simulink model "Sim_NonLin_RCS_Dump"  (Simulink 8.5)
settings: Solver=ode45  StartTime=0.0  StopTime=25*60  FixedStep=Ts  RelTol=1e-3
InitFcn:
  | start2
StopFcn:
  | Pl
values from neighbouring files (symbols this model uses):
  Ave = [    [vehicle_flex34.m]    (also in vehicle_rigid.m)
  Bve = [    [vehicle_flex34.m]    (also in vehicle_rigid.m)
  CB2L = [cpsi, -cphi*spsi,  sphi*spsi;          0,    cphi,      -sphi;          0,    sphi*cpsi,  cphi*cpsi]/cpsi    [Rigbod_Dynam_LVLH.m]    (also in start.m = eye(3); start2.m = eye(3); start3.m = eye(3); start1.m = eye(3))
  com_dir = com_dir/sqrt(com_dir'*com_dir)    [start.m]    (also in start2.m; start3.m; start1.m)
  Cve = [    [vehicle_flex34.m]    (also in vehicle_rigid.m)
  d2r = pi/180    (= 0.0174532925199)    [start.m]    (also in start2.m; start3.m; Dead_Band_DF.m; start1.m)
  Dve = [    [vehicle_flex34.m]    (also in vehicle_rigid.m)
  ini = [wbo; atto; Hco]    [start.m]    (also in start2.m; start3.m; start1.m)
  KshR = 2*Wdot_Lim_RCS/WlimR    [start.m]    (also in start2.m; start3.m; start1.m)
  nt = 12    [start.m]    (also in start2.m; start3.m; start1.m)
  r2d = 180/pi    (= 57.2957795131)    [start.m]    (also in start2.m; start3.m; start1.m)
  thecmd = 20    [start.m]    (also in start2.m; start3.m; start1.m = 0.1)
  Wdot_Lim_RCS = 0.02*d2r    (= 0.000349065850399)    [start.m]    (also in start2.m; start3.m; start1.m)
  Wlim_RCS = 0.6*d2r    (= 0.010471975512)    [start.m]    (also in start2.m; start3.m; start1.m)
  wo = 0.0011    [start.m]    (also in start2.m; start3.m; start1.m)
undefined symbols (not defined in the file or in its folder): Mom_Dump, Phase_Plane, Rigbod_Dynam_LVLH, Wlim

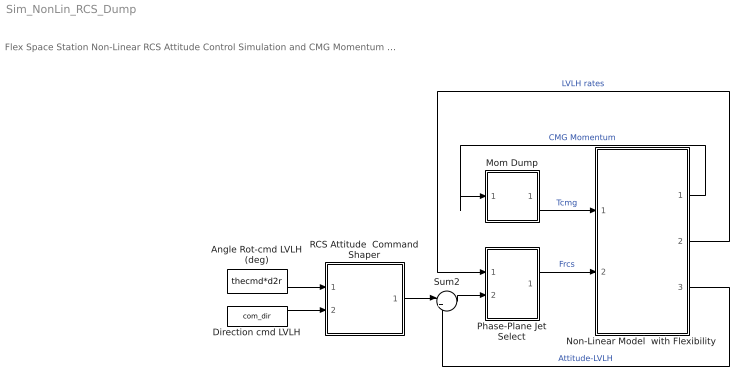
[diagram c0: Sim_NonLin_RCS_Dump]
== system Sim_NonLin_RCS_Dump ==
  note: Flex Space Station Non-Linear RCS Attitude Control Simulation and CMG Momentum Desaturation Mode using RCS
  Angle Rot-cmd LVLH (deg) : Constant  Value=thecmd*d2r
  Direction cmd LVLH : Constant  Value=com_dir
  Mom Dump : Subsystem
  Non-Linear Model  with Flexibility : Subsystem
  Phase-Plane Jet Select : Subsystem
  RCS Attitude  Command Shaper : Subsystem
  Sum2 : Sum  Inputs=|+-
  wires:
  Non-Linear Model  with Flexibility/3(atti) -> Sum2/2  "Attitude-LVLH"
  Non-Linear Model  with Flexibility/1(Hcmg) -> Mom Dump/1(Hcmg)  "CMG Momentum"
  Sum2/1 -> Phase-Plane Jet Select/2(atter)
  Non-Linear Model  with Flexibility/2(w-lv) -> Phase-Plane Jet Select/1(rater)  "LVLH rates"
  Direction cmd LVLH/1 -> RCS Attitude  Command Shaper/2(dir)
  Angle Rot-cmd LVLH (deg)/1 -> RCS Attitude  Command Shaper/1(cmd)
  RCS Attitude  Command Shaper/1(att-cmd) -> Sum2/1
  Phase-Plane Jet Select/1(f(i)) -> Non-Linear Model  with Flexibility/2(Frcs)  "Frcs"
  Mom Dump/1(Tq) -> Non-Linear Model  with Flexibility/1(Tcmg)  "Tcmg"

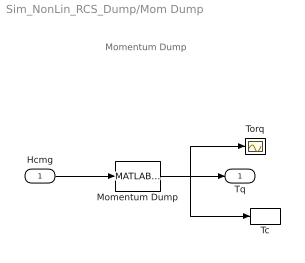
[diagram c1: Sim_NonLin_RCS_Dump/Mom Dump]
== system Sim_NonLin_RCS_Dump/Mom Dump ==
  note: Momentum Dump
  Hcmg : Inport  PortDimensions=3
  Momentum Dump : MATLABFcn  MATLABFcn=Mom_Dump( u(1:3) )  OutputDimensions=3
  Tc : ToWorkspace  VariableName=Tcmg  SampleTime=-1
  Torq : Scope
  Tq : Outport
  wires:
  Momentum Dump/1 -> Tc/1, Torq/1, Tq/1
  Hcmg/1 -> Momentum Dump/1

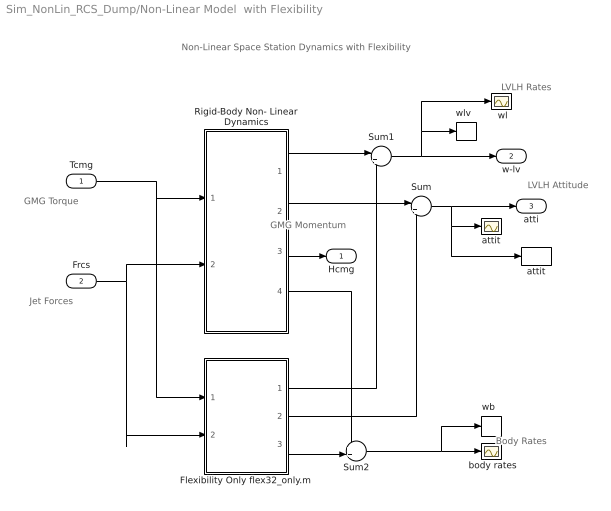
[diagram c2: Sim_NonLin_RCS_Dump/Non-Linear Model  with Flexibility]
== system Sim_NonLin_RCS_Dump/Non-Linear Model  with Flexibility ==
  note: Non-Linear Space Station Dynamics with Flexibility
  note: GMG Torque
  note: Jet Forces
  note: LVLH Rates
  note: LVLH Attitude
  note: Body Rates
  note: GMG Momentum
  Tcmg : Inport
  Frcs : Inport  Port=2
  " attit " : Scope
  " body rates" : Scope
  " wl" : Scope
  Flexibility Only flex32_only.m : Subsystem
  Rigid-Body Non- Linear Dynamics : Subsystem
  Sum : Sum  Inputs=|++
  Sum1 : Sum  Inputs=|++
  Sum2 : Sum  Inputs=++|
  attit : ToWorkspace  VariableName=theta  SampleTime=-1
  "wb  " : ToWorkspace  VariableName=wb  SampleTime=-1
  "wlv  " : ToWorkspace  VariableName=wl  SampleTime=-1
  Hcmg : Outport
  w-lv : Outport  Port=2
  atti : Outport  Port=3
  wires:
  Frcs/1 -> Rigid-Body Non- Linear Dynamics/2(Frcs), Flexibility Only flex32_only.m/2(Frcs)
  Rigid-Body Non- Linear Dynamics/2(atti-lv) -> Sum/1
  Flexibility Only flex32_only.m/2(att) -> Sum/2
  Sum/1 -> atti/1, " attit "/1, attit/1
  Sum1/1 -> w-lv/1, "wlv  "/1, " wl"/1
  Tcmg/1 -> Rigid-Body Non- Linear Dynamics/1(Tcmg), Flexibility Only flex32_only.m/1(Tcmg)
  Rigid-Body Non- Linear Dynamics/1(w-lv) -> Sum1/1
  Flexibility Only flex32_only.m/1(wbf) -> Sum1/2
  Flexibility Only flex32_only.m/3(wb) -> Sum2/2
  Rigid-Body Non- Linear Dynamics/4(wb) -> Sum2/1
  Sum2/1 -> " body rates"/1, "wb  "/1
  Rigid-Body Non- Linear Dynamics/3(Hcmg) -> Hcmg/1

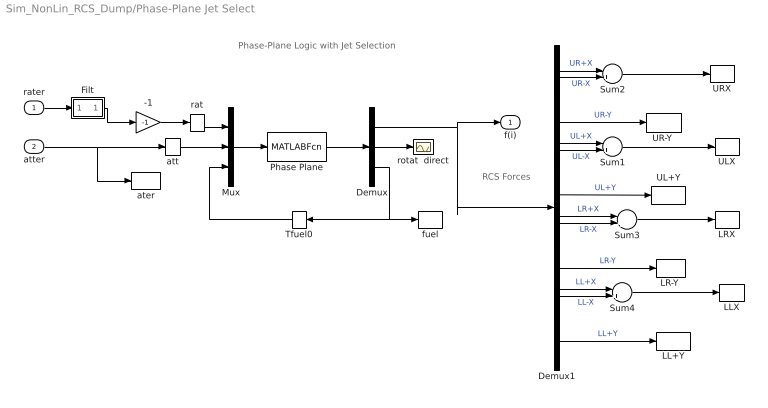
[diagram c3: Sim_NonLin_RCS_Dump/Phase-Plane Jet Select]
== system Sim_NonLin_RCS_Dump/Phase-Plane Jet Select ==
  note: RCS Forces
  note: Phase-Plane Logic with Jet Selection
  rater : Inport
  atter : Inport  Port=2
  -1 : Gain  Gain=-1
  Demux : Demux  Outputs=[nt, 3,1]
  Demux1 : Demux  Outputs=nt
  Filt : Subsystem
  LL+Y : ToWorkspace  VariableName=LLPY  SampleTime=-1
  LLX : ToWorkspace  VariableName=LLX  SampleTime=-1
  "LR-Y " : ToWorkspace  VariableName=LRNY  SampleTime=-1
  LRX : ToWorkspace  VariableName=LRX  SampleTime=-1
  Mux : Mux  Inputs="[3  3  1]"
  Phase Plane : MATLABFcn  MATLABFcn=Phase_Plane( u(1:3), u(4:6), u(7) )  OutputDimensions=nt + 4
  Sum{1..4} (4 alike) : Sum  Inputs=|++
  Tfuel0 : Memory
  UL+Y : ToWorkspace  VariableName=ULPY  SampleTime=-1
  ULX : ToWorkspace  VariableName=ULX  SampleTime=-1
  "UR-Y " : ToWorkspace  VariableName=URNY  SampleTime=-1
  URX : ToWorkspace  VariableName=URX  SampleTime=-1
  ater : ToWorkspace  VariableName=atter  SampleTime=-1
  att : Memory
  fuel : ToWorkspace  VariableName=Fuel  SampleTime=-1
  rat : Memory
  rotat  direct : Scope
  f(i) : Outport
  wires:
  -1/1 -> rat/1
  Demux1/9 -> "LR-Y "/1  "LR-Y"
  Demux1/12 -> LL+Y/1  "LL+Y"
  Demux1/6 -> UL+Y/1  "UL+Y"
  Demux1/3 -> "UR-Y "/1  "UR-Y"
  Sum4/1 -> LLX/1
  Sum3/1 -> LRX/1
  Sum1/1 -> ULX/1
  Demux1/11 -> Sum4/2  "LL-X"
  Demux1/10 -> Sum4/1  "LL+X"
  Demux1/8 -> Sum3/2  "LR-X"
  Demux1/7 -> Sum3/1  "LR+X"
  Demux1/5 -> Sum1/2  "UL-X"
  Demux1/4 -> Sum1/1  "UL+X"
  Sum2/1 -> URX/1
  Demux1/2 -> Sum2/2  "UR-X"
  Demux1/1 -> Sum2/1  "UR+X"
  rat/1 -> Mux/1
  Mux/1 -> Phase Plane/1
  Phase Plane/1 -> Demux/1
  Tfuel0/1 -> Mux/3
  Demux/1 -> Demux1/1, f(i)/1
  Demux/2 -> rotat  direct/1
  atter/1 -> ater/1, att/1
  att/1 -> Mux/2
  Demux/3 -> fuel/1, Tfuel0/1
  rater/1 -> Filt/1(I)
  Filt/1(O) -> -1/1

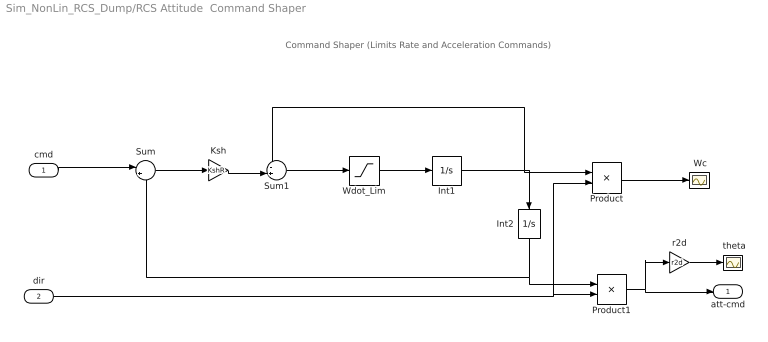
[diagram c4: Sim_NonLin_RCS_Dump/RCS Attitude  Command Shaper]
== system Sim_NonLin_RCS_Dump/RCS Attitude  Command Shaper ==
  note: Command Shaper (Limits Rate and Acceleration Commands)
  cmd : Inport  PortDimensions=1
  dir : Inport  Port=2  PortDimensions=3
  " Wc" : Scope
  " theta" : Scope
  Int1 : Integrator  LimitOutput=on  UpperSaturationLimit=Wlim_RCS  LowerSaturationLimit=-Wlim_RCS
  Int2 : Integrator  UpperSaturationLimit=Wlim  LowerSaturationLimit=-Wlim
  Ksh : Gain  Gain=KshR
  Product : Product
  Product1 : Product
  Sum : Sum  Inputs=|+-
  Sum1 : Sum  Inputs=-+|
  Wdot_Lim : Saturate  UpperLimit=Wdot_Lim_RCS  LowerLimit=-Wdot_Lim_RCS
  r2d : Gain  Gain=r2d
  att-cmd : Outport  PortDimensions=3
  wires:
  Wdot_Lim/1 -> Int1/1
  Sum1/1 -> Wdot_Lim/1
  Int1/1 -> Product/1, Sum1/1, Int2/1
  Sum/1 -> Ksh/1
  Ksh/1 -> Sum1/2
  Int2/1 -> Sum/2, Product1/1
  cmd/1 -> Sum/1
  dir/1 -> Product/2, Product1/2
  r2d/1 -> " theta"/1
  Product/1 -> " Wc"/1
  Product1/1 -> att-cmd/1, r2d/1

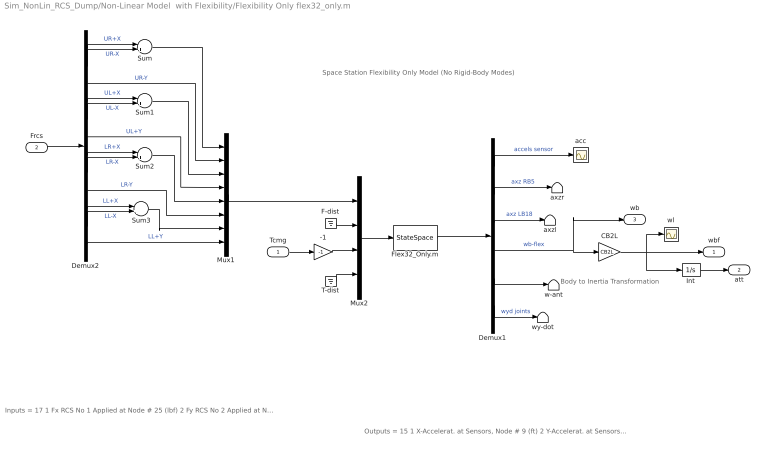
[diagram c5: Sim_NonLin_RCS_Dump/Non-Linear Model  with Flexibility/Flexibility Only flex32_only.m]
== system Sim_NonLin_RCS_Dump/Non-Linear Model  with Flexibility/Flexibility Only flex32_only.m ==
  note: Outputs = 15 1 X-Accelerat. at Sensors, Node # 9 (ft) 2 Y-Accelerat. at Sensors, Node # 9 (ft) 3 Z-Accelerat. at Sensors, Node # 9 (ft) 4 X-Accelerat. at Right Boom End, Node # 5 (ft) 5 Z-Accelerat. at Right Boom End, Node # 5 (ft) 6 X-Accelerat. at Left Boom End, Node # 18 (ft) 7 Z-Accelerat. at Left Boom End, Node # 18 (ft) 8 X-Rot. Rate at Sensors, Node # 9 (radian) 9 Y-Rot. Rate at Sensors, Node # 9 (radian) 10 Z-Rot. Rate at Sensors, Node # 9 (radian) 11 X-Rot. Rate at Antena Bot-Left, Node # 24 (radian) 12 Y-Rot. Rate at Antena Bot-Left, Node # 24 (radian) 13 Z-Rot. Rate at Antena Bot-Left, Node # 24 (radian) 14 Y-Rot.Accel. at Right Joint, Node # 7 (radian) 15 Y-Rot.Accel. at Left Joint, Node # 16 (radian)
  note: Inputs = 17 1 Fx RCS No 1 Applied at Node # 25 (lbf) 2 Fy RCS No 2 Applied at Node # 25 (lbf) 3 Fx RCS No 3 Applied at Node # 26 (lbf) 4 Fy RCS No 4 Applied at Node # 26 (lbf) 5 Fx RCS No 5 Applied at Node # 27 (lbf) 6 Fy RCS No 6 Applied at Node # 27 (lbf) 7 Fx RCS No 7 Applied at Node # 28 (lbf) 8 Fy RCS No 8 Applied at Node # 28 (lbf) 9 Fx Disturb. No 9 at Node # 21 (lbf) 10 Fy Disturb. No 10 at Node # 21 (lbf) 11 Fz Disturb. No 11 at Node # 21 (lbf) 12 Torq-x No 1 CMG Applied at Node # 10 (ft-lb) 13 Torq-y No 2 CMG Applied at Node # 10 (ft-lb) 14 Torq-z No 3 CMG Applied at Node # 10 (ft-lb) 15 Torq-x No 4 Gimbal Dist. at Node # 1 (ft-lb) 16 Torq-y No 5 Gimbal Dist. at Node # 1 (ft-lb) 17 Torq-z No 6 Gimbal Dist. at Node # 1 (ft-lb)
  note: Space Station Flexibility Only Model (No Rigid-Body Modes)
  note: Body to Inertia Transformation
  Tcmg : Inport
  Frcs : Inport  Port=2
  -1 : Gain  Gain=-1
  CB2L : Gain  Gain=CB2L  Multiplication=Matrix(K*u)
  Demux1 : Demux  Outputs=[3, 2, 2, 3, 3, 2]
  Demux2 : Demux  Outputs=12
  F-dist : Ground
  Flex32_Only.m : StateSpace  A=Ave  B=Bve  C=Cve  D=Dve  X0=0
  Int : Integrator
  Mux1 : Mux  Inputs=8
  Mux2 : Mux  Inputs=[8, 3, 3, 3]
  Sum{,1..3} (4 alike) : Sum  Inputs=|+-
  T-dist : Ground
  acc : Scope
  axzl : Terminator
  axzr : Terminator
  w-ant : Terminator
  wl : Scope
  wy-dot : Terminator
  wbf : Outport
  att : Outport  Port=2
  wb : Outport  Port=3
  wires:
  Demux1/6 -> wy-dot/1  "wyd joints"
  Demux1/5 -> w-ant/1
  T-dist/1 -> Mux2/4
  F-dist/1 -> Mux2/2
  Demux1/3 -> axzl/1  "axz LB18"
  Demux1/2 -> axzr/1  "axz RB5"
  Tcmg/1 -> -1/1
  Demux1/4 -> CB2L/1, wb/1  "wb-flex"
  Demux1/1 -> acc/1  "accels sensor"
  Flex32_Only.m/1 -> Demux1/1
  Mux2/1 -> Flex32_Only.m/1
  Mux1/1 -> Mux2/1
  Frcs/1 -> Demux2/1
  Demux2/6 -> Mux1/4  "UL+Y"
  Demux2/9 -> Mux1/6  "LR-Y"
  Demux2/12 -> Mux1/8  "LL+Y"
  Demux2/3 -> Mux1/2  "UR-Y"
  Demux2/1 -> Sum/1  "UR+X"
  Demux2/2 -> Sum/2  "UR-X"
  Sum/1 -> Mux1/1
  Demux2/4 -> Sum1/1  "UL+X"
  Demux2/5 -> Sum1/2  "UL-X"
  Sum1/1 -> Mux1/3
  Demux2/7 -> Sum2/1  "LR+X"
  Demux2/8 -> Sum2/2  "LR-X"
  Demux2/10 -> Sum3/1  "LL+X"
  Demux2/11 -> Sum3/2  "LL-X"
  Sum3/1 -> Mux1/7
  Sum2/1 -> Mux1/5
  Int/1 -> att/1
  -1/1 -> Mux2/3
  CB2L/1 -> wl/1, wbf/1, Int/1

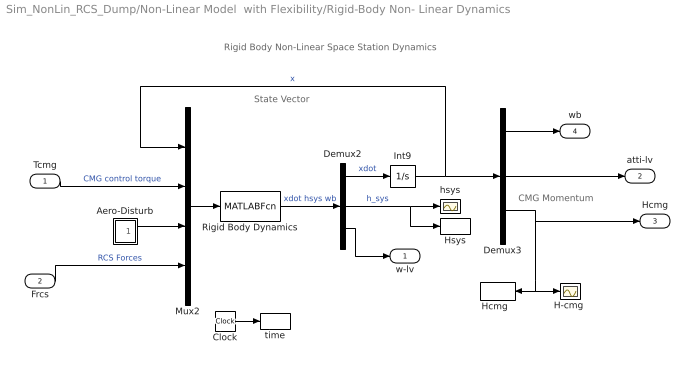
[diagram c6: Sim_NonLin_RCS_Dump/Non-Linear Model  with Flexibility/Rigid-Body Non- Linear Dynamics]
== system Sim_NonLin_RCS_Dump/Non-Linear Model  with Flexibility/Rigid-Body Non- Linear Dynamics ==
  note: CMG Momentum
  note: State Vector
  note: Rigid Body Non-Linear Space Station Dynamics
  Tcmg : Inport  PortDimensions=3
  Frcs : Inport  Port=2  PortDimensions=nt
  Aero-Disturb : Subsystem
  Clock : Clock
  Demux2 : Demux  Outputs=[9,3,3]
  Demux3 : Demux  Outputs=[3,3,3]
  "H-cmg " : Scope
  "Hcmg  " : ToWorkspace  VariableName=Hcmg  SampleTime=-1
  Hsys : ToWorkspace  VariableName=Hsys  SampleTime=-1
  Int9 : Integrator  InitialCondition=ini
  Mux2 : Mux  Inputs=[9, 3, 3, nt]
  Rigid Body Dynamics : MATLABFcn  MATLABFcn=Rigbod_Dynam_LVLH( u(1:9), u(10:12), u(13:15), u(16:15+nt) )  OutputDimensions=15
  hsys : Scope
  time : ToWorkspace  VariableName=time  SampleTime=-1
  w-lv : Outport
  atti-lv : Outport  Port=2
  Hcmg : Outport  Port=3
  wb : Outport  Port=4
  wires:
  Mux2/1 -> Rigid Body Dynamics/1
  Clock/1 -> time/1
  Frcs/1 -> Mux2/4  "RCS Forces"
  Demux3/3 -> Hcmg/1, "H-cmg "/1, "Hcmg  "/1
  Demux3/2 -> atti-lv/1
  Demux2/2 -> Hsys/1, hsys/1  "h_sys"
  Demux2/3 -> w-lv/1
  Tcmg/1 -> Mux2/2  "CMG control torque"
  Int9/1 -> Mux2/1, Demux3/1  "x"
  Demux2/1 -> Int9/1  "xdot"
  Rigid Body Dynamics/1 -> Demux2/1  "xdot hsys wb"
  Aero-Disturb/1(Td) -> Mux2/3
  Demux3/1 -> wb/1

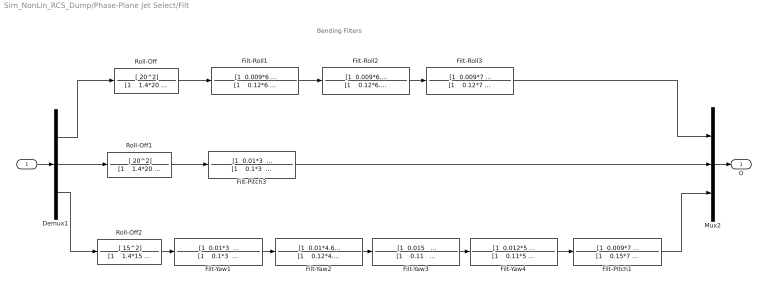
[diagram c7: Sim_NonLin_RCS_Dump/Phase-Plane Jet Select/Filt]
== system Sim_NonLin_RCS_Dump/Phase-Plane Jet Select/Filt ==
  note: Bending Filters
  I : Inport
  Demux1 : Demux  Outputs=3
  Filt-Pitch1 : TransferFcn  Numerator="[1  0.009*7   6.83^2]"  Denominator="[1    0.15*7    6.83^2]"
  Filt-Pitch3 : TransferFcn  Numerator="[1  0.01*3   3.07^2]"  Denominator="[1    0.1*3    3.07^2]"
  Filt-Roll1 : TransferFcn  Numerator="[1  0.009*6   5.85^2]"  Denominator="[1    0.12*6    5.85^2]"
  Filt-Roll2 : TransferFcn  Numerator="[1  0.009*6.4   6.46^2]"  Denominator="[1    0.12*6.4    6.46^2]"
  Filt-Roll3 : TransferFcn  Numerator="[1  0.009*7   7.51^2]"  Denominator="[1    0.12*7    7.51^2]"
  Filt-Yaw1 : TransferFcn  Numerator="[1  0.01*3   3.07^2]"  Denominator="[1    0.1*3    3.07^2]"
  Filt-Yaw2 : TransferFcn  Numerator="[1  0.01*4.6   4.6^2]"  Denominator="[1    0.12*4.6    4.6^2]"
  Filt-Yaw3 : TransferFcn  Numerator="[1  0.015   1.14^2]"  Denominator="[1    0.11    1.14^2]"
  Filt-Yaw4 : TransferFcn  Numerator="[1  0.012*5   5.21^2]"  Denominator="[1    0.11*5    5.21^2]"
  Mux2 : Mux  Inputs=3
  Roll-Off : TransferFcn  Numerator=[ 20^2]  Denominator="[1    1.4*20    20^2]"
  Roll-Off1 : TransferFcn  Numerator=[ 20^2]  Denominator="[1    1.4*20    20^2]"
  Roll-Off2 : TransferFcn  Numerator=[ 15^2]  Denominator="[1    1.4*15    15^2]"
  O : Outport
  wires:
  I/1 -> Demux1/1
  Mux2/1 -> O/1
  Demux1/1 -> Roll-Off/1
  Demux1/3 -> Roll-Off2/1
  Demux1/2 -> Roll-Off1/1
  Roll-Off/1 -> Filt-Roll1/1
  Roll-Off2/1 -> Filt-Yaw1/1
  Roll-Off1/1 -> Filt-Pitch3/1
  Filt-Roll1/1 -> Filt-Roll2/1
  Filt-Roll2/1 -> Filt-Roll3/1
  Filt-Roll3/1 -> Mux2/1
  Filt-Pitch3/1 -> Mux2/2
  Filt-Yaw1/1 -> Filt-Yaw2/1
  Filt-Yaw2/1 -> Filt-Yaw3/1
  Filt-Yaw3/1 -> Filt-Yaw4/1
  Filt-Yaw4/1 -> Filt-Pitch1/1
  Filt-Pitch1/1 -> Mux2/3

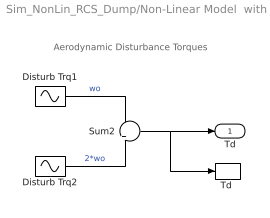
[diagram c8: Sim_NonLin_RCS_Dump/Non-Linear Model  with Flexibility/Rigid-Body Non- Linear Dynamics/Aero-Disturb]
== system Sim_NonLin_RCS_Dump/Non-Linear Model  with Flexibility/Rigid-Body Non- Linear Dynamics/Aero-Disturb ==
  note: Aerodynamic Disturbance Torques
  Disturb Trq1 : Sin  Amplitude=[1, 3, 1]  Bias="[1  8  1]"  Frequency=[wo, wo, wo]  SampleTime=0
  Disturb Trq2 : Sin  Amplitude=[1, 1, 1]*0.5  Frequency=[wo, wo, wo]*2  SampleTime=0
  Sum2 : Sum  Inputs=+|+
  "Td " : ToWorkspace  VariableName=Td  SampleTime=-1
  Td : Outport
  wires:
  Disturb Trq2/1 -> Sum2/2  "2*wo"
  Sum2/1 -> "Td "/1, Td/1
  Disturb Trq1/1 -> Sum2/1  "wo"
